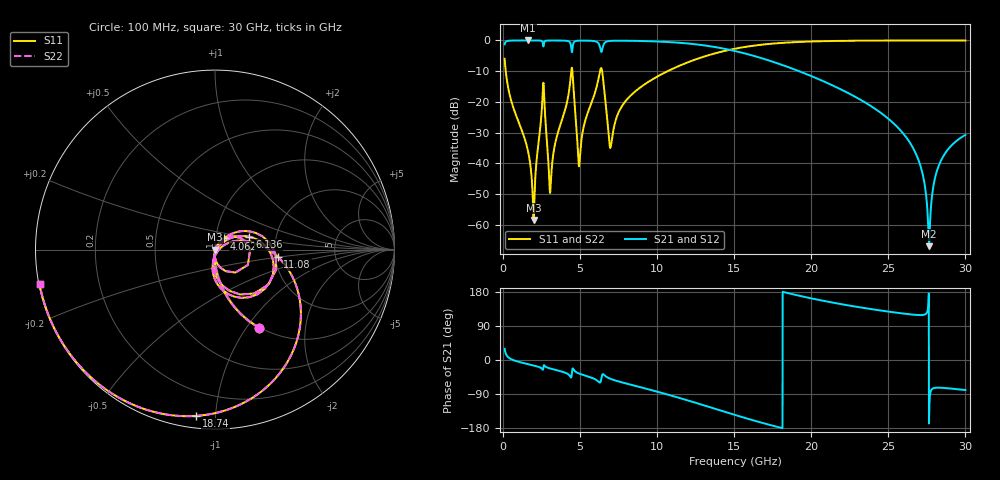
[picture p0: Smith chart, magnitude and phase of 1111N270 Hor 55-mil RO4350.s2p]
# GHz S MA R 50
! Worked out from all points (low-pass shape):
!   3201 points, 100 MHz to 30 GHz, reference 50 ohm
!   highest |S21| = -0.01 dB at 1.632 GHz (marker M1); lowest = -67.0 dB at 27.65 GHz (marker M2)
!   |S21| within 3 dB of the highest: start of sweep to 4.438 GHz; 6.434 GHz to 14.65 GHz (8.214 GHz wide, 77.9 % of centre)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
!   lowest |S11| = -58.4 dB at 1.978 GHz (marker M3), VSWR 1.00, Z = 50.1 - j0.0421 ohm
!   |S11| at or under -10 dB: 174.1 MHz to 4.422 GHz (4.248 GHz wide, 185 % of centre); 4.497 GHz to 6.289 GHz (1.793 GHz wide, 33.2 % of centre); 6.427 GHz to 10.68 GHz (4.257 GHz wide, 49.8 % of centre)
!   |S22| runs from -58.4 to 0.0 dB; largest |S21 - S12| = 0
!   S11 on the Smith chart (normalised r, x): 100 MHz: 0.99, -1.16; 4.062 GHz: 1.10, +0.14; 6.136 GHz: 1.46, +0.22; 11.08 GHz: 2.07, -0.19; 18.74 GHz: 0.06, -0.89; 30 GHz: 0.00, -0.10
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0.1  0.5032 -60.5  0.8639 29.5  0.8639 29.5  0.5032 -60.5
1.632375  0.01524 -97.8  0.9988 -11.1  0.9988 -11.1  0.01524 -97.8
1.978094  0.001197 -20.5  0.9986 -14.5  0.9986 -14.5  0.001197 -20.5
2.56675  0.1293 35.1  0.9294 -25.3  0.9294 -25.3  0.1293 35.1
3.071312  0.003666 8.8  0.9965 -22.5  0.9965 -22.5  0.003666 8.8
4.06175  0.08016 51.0  0.9894 -34.1  0.9894 -34.1  0.08016 51.0
4.463531  0.3602 -25.8  0.6428 -35.9  0.6428 -35.9  0.3602 -25.8
4.865312  0.01386 -75.5  0.9889 -34.6  0.9889 -34.6  0.01386 -75.5
5.089563  0.02435 36.4  0.9926 -38.0  0.9926 -38.0  0.02435 36.4
6.136063  0.205 20.4  0.9284 -55.2  0.9284 -55.2  0.205 20.4
6.435062  0.3064 -61.4  0.709 -39.1  0.709 -39.1  0.3064 -61.4
6.986344  0.01841 -21.0  0.9831 -49.9  0.9831 -49.9  0.01841 -21.0
10.06978  0.263 4.7  0.9593 -84.3  0.9593 -84.3  0.263 4.7
11.07891  0.3524 -6.5  0.93 -95.8  0.93 -95.8  0.3524 -6.5
15.05  0.7332 -55.4  0.6717 -145.0  0.6717 -145.0  0.7332 -55.4
18.74078  0.9323 -96.4  0.3496 174.1  0.3496 174.1  0.9323 -96.4
20.03956  0.9614 -108.2  0.2603 162.3  0.2603 162.3  0.9614 -108.2
25.01978  0.9954 -143.2  0.05261 127.6  0.05261 127.6  0.9954 -143.2
26.89787  0.9968 -153.6  0.01233 118.8  0.01233 118.8  0.9968 -153.6
27.64538  0.9969 -157.5  0.0004474 -149.1  0.0004474 -149.1  0.9969 -157.5
28.33681  0.9969 -160.9  0.01002 -73.1  0.01002 -73.1  0.9969 -160.9
30  0.9965 -168.8  0.02898 -79.3  0.02898 -79.3  0.9965 -168.8
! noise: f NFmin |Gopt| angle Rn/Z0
0.1  0.0007155  0.7521  2.112  0.0005821
3.417  0.01265  0.5736  24.69  0.005146
6.743  0.0645  0.8162  47.88  0.06142
10.06  0.02893  0.5145  65.36  0.007672
13.39  0.0403  0.5577  80.91  0.01002
16.7  0.06287  0.6641  97.34  0.01646
20.03  0.1135  0.7939  115.8  0.03322
23.35  0.2654  0.9065  134.7  0.09359
26.67  1.604  0.9836  152.6  1.287
30  0.9239  0.9713  168.6  0.07357
